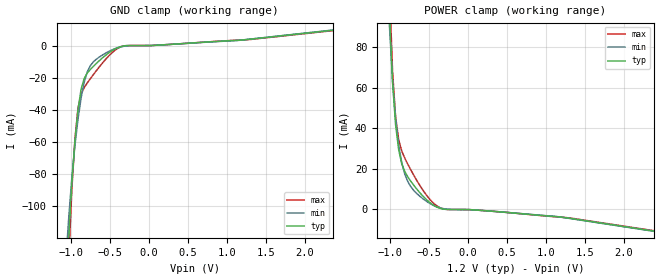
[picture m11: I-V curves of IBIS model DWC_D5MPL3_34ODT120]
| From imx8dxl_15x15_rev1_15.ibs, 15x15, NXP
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[Model] DWC_D5MPL3_34ODT120
Model_type   Input
Polarity   Non-Inverting
Enable   Active-High
C_comp   1.276pF   1.192pF   1.376pF
C_comp_power_clamp   301.771fF   275.484fF   323.862fF
C_comp_gnd_clamp 964.284fF   900.446fF   1.045pF
Vinh = 868.000mV
Vinl = 598.000mV
[Model Spec]
D_overshoot_ampl_h 0.35 NA   NA
D_overshoot_ampl_l 0.35 NA   NA
D_overshoot_area_l 100.000p NA   NA
D_overshoot_area_h 100.000p NA   NA
[Receiver Thresholds]
Vth = 733.000mV
Vth_min = 721.000mV
Vth_max = 745.000mV
Vinh_ac = 135.000mV
Vinh_dc = 100.000mV
Vinl_ac = -135.000mV
Vinl_dc = -100.000mV
Tslew_ac = 5.000ns
Reference_supply Power_clamp_ref
[Temperature Range]   25.000   125.000   -40.000
[Voltage Range]   1.200V   1.140V   1.300V
[GND Clamp Reference]   0.00V   0.00V   0.00V
[C Comp Corner]
| variable   typ   min   max
C_comp 1.276pF   1.376pF   1.192pF
C_comp_pullup 301.771fF   323.862fF   275.484fF
C_comp_pulldown 964.284fF   1.045pF   900.446fF
[POWER Clamp Reference]   1.200V   1.140V   1.300V
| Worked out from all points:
|   GND clamp passes 1 mA (typ) near -0.38 V on its own axis
|   POWER clamp passes 1 mA (typ) near -0.39 V on its own axis
[GND Clamp]
-1.182V   -335.7mA   -251.3mA   -422.9mA
-1.064V   -160.4mA   -134.9mA   -187.2mA
-1.024V   -118.3mA   -105.9mA   -131.3mA
-984.8mV  -84.83mA   -81.72mA   -88.7mA
-945.5mV  -58.88mA   -61.8mA    -57.92mA
-906.1mV  -39.62mA   -45.49mA   -38.71mA
-866.7mV  -27.08mA   -32.47mA   -29.97mA
-787.9mV  -17.05mA   -16.31mA   -23.19mA
-669.7mV  -10.96mA   -8.364mA   -15.45mA
-472.7mV  -3.175mA   -2.682mA   -4.494mA
-315.2mV  -126.8uA   -344.7uA   -87.65uA
2.364V    9.614mA    9.741mA    9.358mA
[Power Clamp]
-1.164V   359.7mA    265.4mA    462.4mA
-1.006V   96.92mA    90.43mA    109.7mA
-966.7mV  62.81mA    63.8mA     68.27mA
-927.3mV  41.78mA    44.77mA    45.59mA
-887.9mV  29.48mA    31.79mA    34.38mA
-848.5mV  22.59mA    23.1mA     28.83mA
-769.7mV  16.02mA    13.65mA    22.28mA
-572.7mV  6.416mA    5.167mA    9.279mA
-415.1mV  1.511mA    1.548mA    2.246mA
-297mV    104.7uA    292.1uA    155.5uA
1.2V      -3.74mA    -3.819mA   -3.843mA
2.382V    -10.67mA   -10.76mA   -10.46mA
